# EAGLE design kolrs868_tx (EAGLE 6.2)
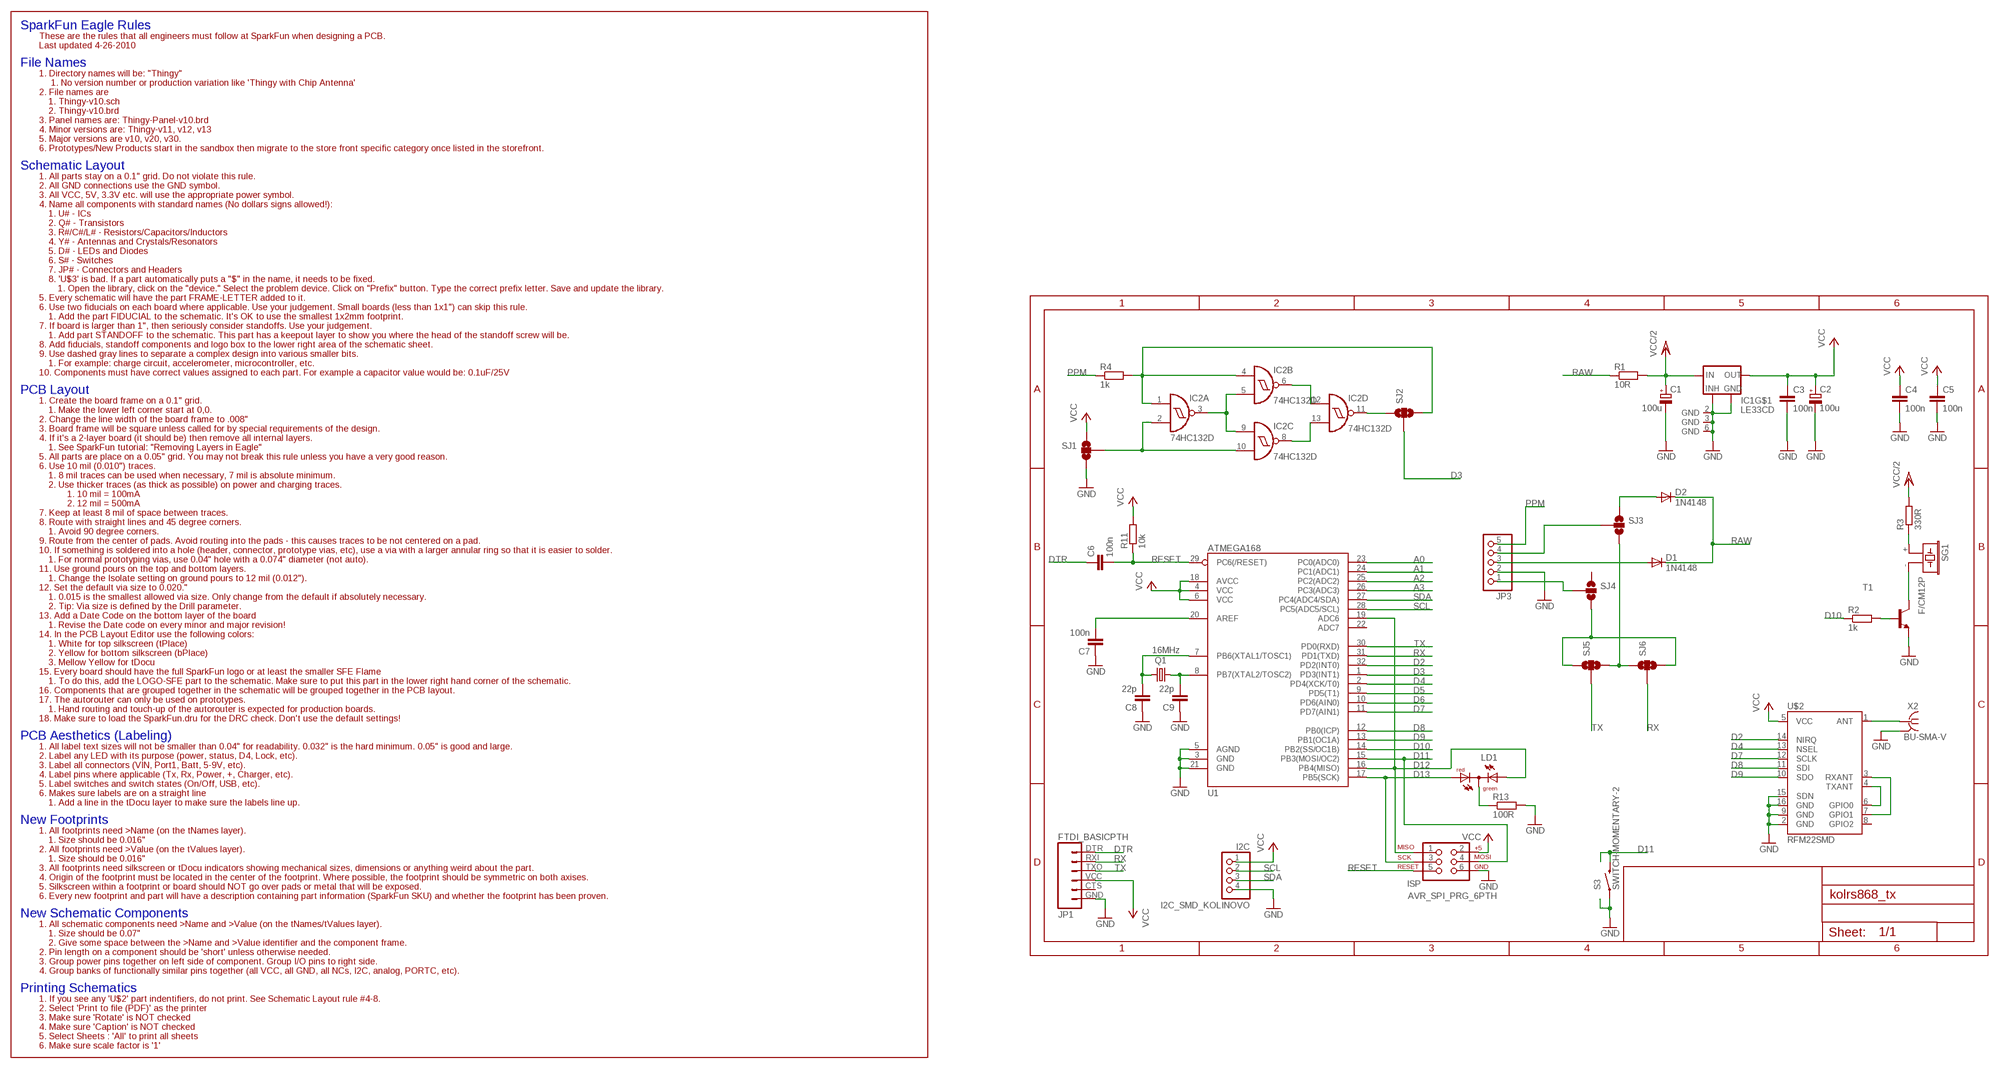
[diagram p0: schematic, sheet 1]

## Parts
C1  100u  CPOL-EUSMCB  [SMC_B]
C2  100u  CPOL-EUSMCB  [SMC_B]
C3  100n  C-EU_KOLIN  [M0805]
C4  100n  C-EU_KOLIN  [M0805]
C5  100n  C-EU_KOLIN  [M0805]
C6  100n  C-EU_KOLIN  [M0805]
C7  100n  C-EU_KOLIN  [M0805]
C8  22p  C-EU_KOLIN  [M0805]
C9  22p  C-EU_KOLIN  [M0805]
D1  1N4148  DIODE-MINIMELF  [MINIMELF]
D2  1N4148  DIODE-MINIMELF  [MINIMELF]
I2C  I2C_SMD_KOLINOVO  [1X04]
IC1  LE33CD  [SO8]
IC2  74HC132D  [SO14]
ISP  AVR_SPI_PRG_6PTH  [2X3]
JP1  FTDI_BASICPTH  [FTDI_BASIC]
JP3  PINHD-1X5  [1X05]
LD1  DUOLED-RG-C  [DUOLED-C-5MM]
Q1  16MHz  CRYSTALHC49UP  [HC49UP]
R1  10R  R-EU_KOLINM0805  [M0805]
R2  1k  R-EU_KOLINM0805  [M0805]
R3  330R  R-EU_KOLINM0805  [M0805]
R4  1k  R-EU_KOLINM0805  [M0805]
R11  10k  R-EU_KOLINM0805  [M0805]
R13  100R  R-EU_KOLINM0805  [M0805]
S3  SWITCH-MOMENTARY-2  [TACTILE_SWITCH_TALL]
SG1  F/CM12P  [F/CM12P]
SJ1  SOLDERJUMPER_2WAYS  [SJ_3]
SJ2  SOLDERJUMPER_2WAYS  [SJ_3]
SJ3  SOLDERJUMPER_2WAYS  [SJ_3]
SJ4  SOLDERJUMPER_2WAYS  [SJ_3]
SJ5  SOLDERJUMPER_2WAYS  [SJ_3]
SJ6  SOLDERJUMPER_2WAYS  [SJ_3]
T1  BC848-NPN-SOT23-BEC  [SOT23-BEC]
U1  ATMEGA168  [TQFP32-08]
U$2  RFM22SMD  [RFM22-XXX-S2]
X2  BU-SMA-V  [BU-SMA-V]

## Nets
A0: U1.23(PC0(ADC0))
A1: U1.24(PC1(ADC1))
A2: U1.25(PC2(ADC2))
A3: U1.26(PC3(ADC3))
D2: U1.32(PD2(INT0)) U$2.14(NIRQ)
D3: SJ2.2 U1.1(PD3(INT1))
D4: U1.2(PD4(XCK/T0)) U$2.13(NSEL)
D5: U1.9(PD5(T1))
D6: U1.10(PD6(AIN0))
D7: U1.11(PD7(AIN1)) U$2.12(SCLK)
D8: U1.12(PB0(ICP)) U$2.11(SDI)
D9: U1.13(PB1(OC1A)) U$2.10(SDO)
D10: R2.1 U1.14(PB2(SS/OC1B))
D11: ISP.4 S3.B2 U1.15(PB3(MOSI/OC2))
D12: ISP.1 LD1.AX(AG) U1.16(PB4(MISO)) U1.19(ADC6)
D13: ISP.3 LD1.AR U1.17(PB5(SCK))
DTR: C6.1 JP1.DTR
GND: C1.- C2.- C3.2 C4.2 C5.2 C7.1 C8.1 C9.1 I2C.4 IC1.2(GND) IC1.3(GND) IC1.5(INHIBIT) IC1.6(GND) IC1.7(GND) ISP.6 JP1.GND JP3.2 R13.2 S3.A2 SJ1.3 T1.E U1.3(GND) U1.5(AGND) U1.21(GND) U$2.2(GND) U$2.9(GND) U$2.15(SDN) U$2.16(GND) X2.2(GND)
N$1: C7.2 U1.20(AREF)
N$2: U$2.4(TXANT) U$2.6(GPIO0)
N$3: U$2.3(RXANT) U$2.7(GPIO1)
N$4: U$2.1(ANT) X2.1
N$5: JP3.1 SJ4.2
N$6: C8.2 Q1.2 U1.7(PB6(XTAL1/TOSC1))
N$7: C9.2 Q1.1 U1.8(PB7(XTAL2/TOSC2))
N$8: LD1.C R13.1
N$10: R2.2 T1.B
N$11: SG1.- T1.C
N$12: R3.1 SG1.+
N$13: D1.A JP3.3
N$14: JP3.4 SJ3.2
N$16: D2.A SJ3.1
N$17: IC2.3(A:O) IC2.5(B:I1) IC2.9(C:I0)
N$18: IC2.11(D:O) SJ2.1
N$19: IC2.2(A:I1) IC2.10(C:I1) SJ1.2
N$20: IC2.8(C:O) IC2.13(D:I1)
N$21: IC2.6(B:O) IC2.12(D:I0)
N$24: IC2.1(A:I0) IC2.4(B:I0) R4.2 SJ2.3
N$25: SJ4.3 SJ5.1 SJ6.3
N$26: SJ3.3 SJ5.3 SJ6.1
PPM: JP3.5 R4.1
RAW: D1.C D2.C R1.1
RESET: C6.2 ISP.5 R11.1 U1.29(PC6(/RESET))
RX: JP1.RXI SJ6.2 U1.31(PD1(TXD))
SCL: I2C.2 U1.28(PC5(ADC5/SCL))
SDA: I2C.3 U1.27(PC4(ADC4/SDA))
TX: JP1.TXO SJ5.2 U1.30(PD0(RXD))
VCC: C2.+ C3.1 C4.1 C5.1 I2C.1 IC1.1(OUT) ISP.2 JP1.VCC R11.2 SJ1.1 U1.4(VCC) U1.6(VCC) U1.18(AVCC) U$2.5(VCC)
VCC/2: C1.+ IC1.8(IN) R1.2 R3.2
Unconnected: JP1.CTS SJ4.1 U1.22(ADC7) U$2.8(GPIO2)

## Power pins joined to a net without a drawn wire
GND: IC2.7(P:GND) X2.3(GND) X2.4(GND) X2.5(GND)
VCC: IC2.14(P:VCC)

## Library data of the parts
C1 C2 = rcl:CPOL-EU: POLARIZED CAPACITOR, European symbol
C3-C9 = PINHEAD_RC:C-EU_KOLIN: CAPACITOR, European symbol
D1 D2 = diode:DIODE-: DIODE
I2C = PINHEAD_RC:I2C_SMD_KOLINOVO: PIN HEADER
IC1 = libstabilizatory:LE33CD: VOLTAGE REGULATOR WITH INHIBIT
IC2 = 74xx-eu:74*132: Quad 2-input NAND schmitt trigger
ISP = SparkFun:AVR_SPI_PRG_6: AVR ISP 6 Pin This is the reduced ISP connector for AVR programming. Common on Arduino. This footprint will take up less PCB space and can be used with a 10-pin to 6-pin adapter such as SKU: BOB-08508
JP1 = SparkFun:FTDI_BASIC: FTDI Basic: 3.3V and 5V
JP3 = pinhead:PINHD-1X5: PIN HEADER
LD1 = led:DUOLED-RG-C: DUO LED 2 colors (red/green), 5 mm, round, common Cathode www.ligitek.com or other producers.
Q1 = crystal:CRYSTAL: CRYSTAL; OC_FARNELL: unknown; OC_NEWARK: unknown
R1-R4 R11 R13 = PINHEAD_RC:R-EU_KOLIN: RESISTOR, European symbol
S3 = SparkFun:SWITCH-MOMENTARY-2
SG1 = buzzer:F/CM12P: BUZZER
SJ1-SJ6 = SparkFun:SOLDERJUMPER_2WAY: Solder Jumper 2 way solder jumper
T1 = transistor:*-NPN-: NPN Transistror BF959 corrected 2008.03.06
U1 = SparkFun:ATMEGA168
U$2 = SparkFun:RFM22: Description: The RFM22 is a low-power, low cost radio that is capable of operating in the 434MHz and 900MHz open bands. It's frequency is software defined and there are some very good libraries written for it.
X2 = con-coax:BU-SMA-V: FEMALE SMA CONNECTOR Radiall distributor RS 112-3794; OC_FARNELL: unknown; OC_NEWARK: unknown

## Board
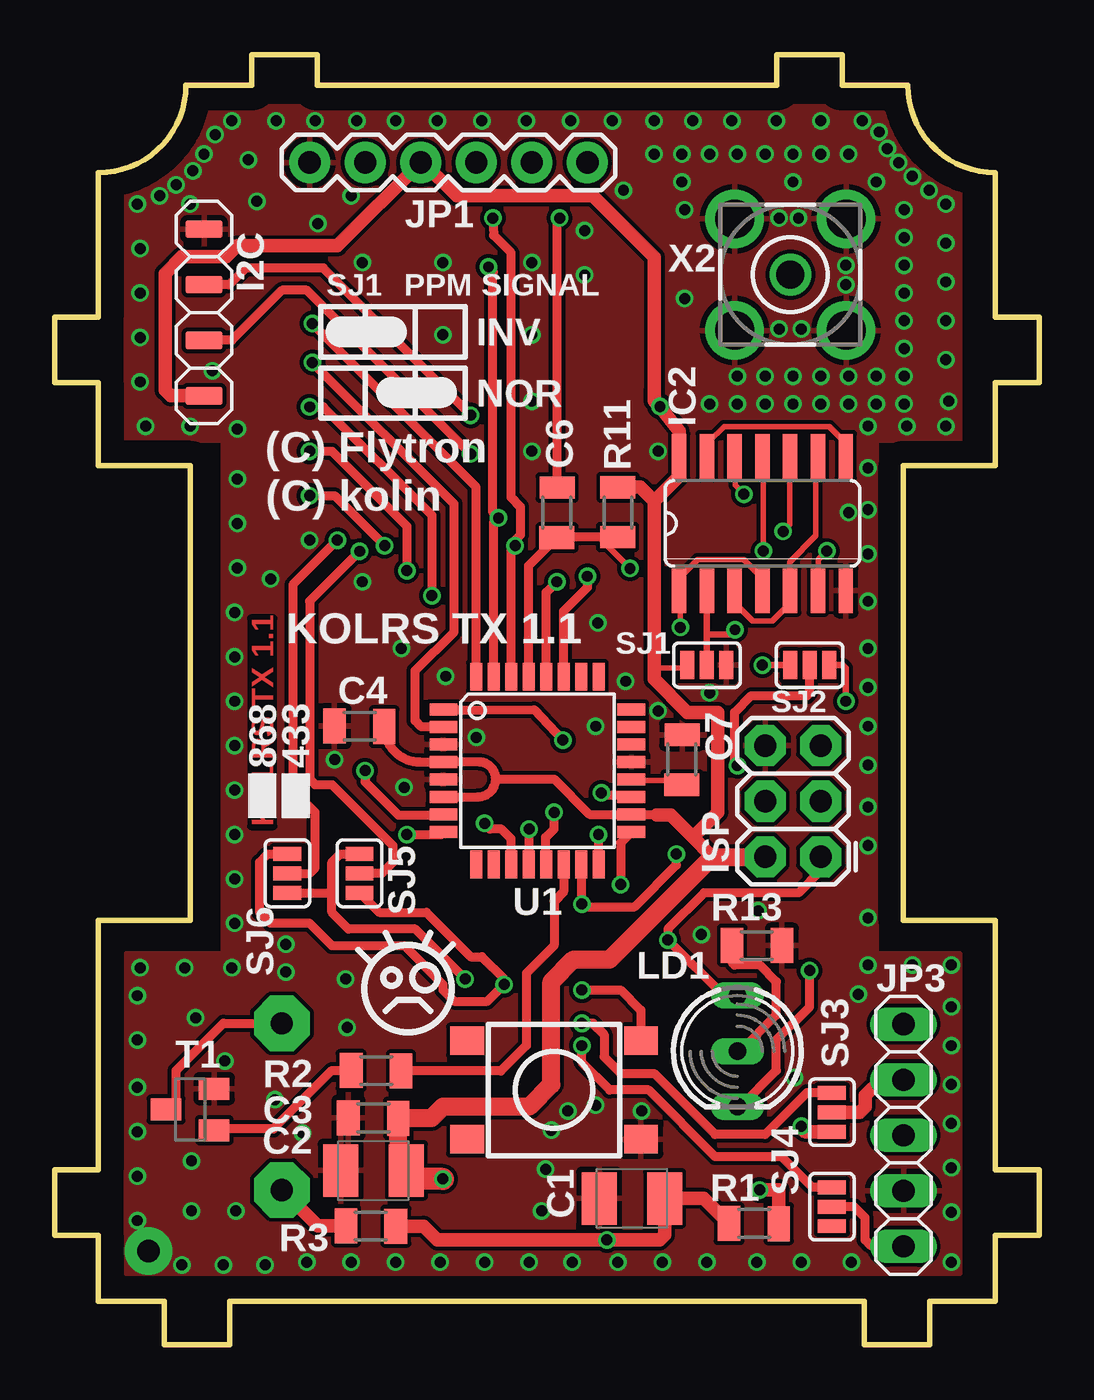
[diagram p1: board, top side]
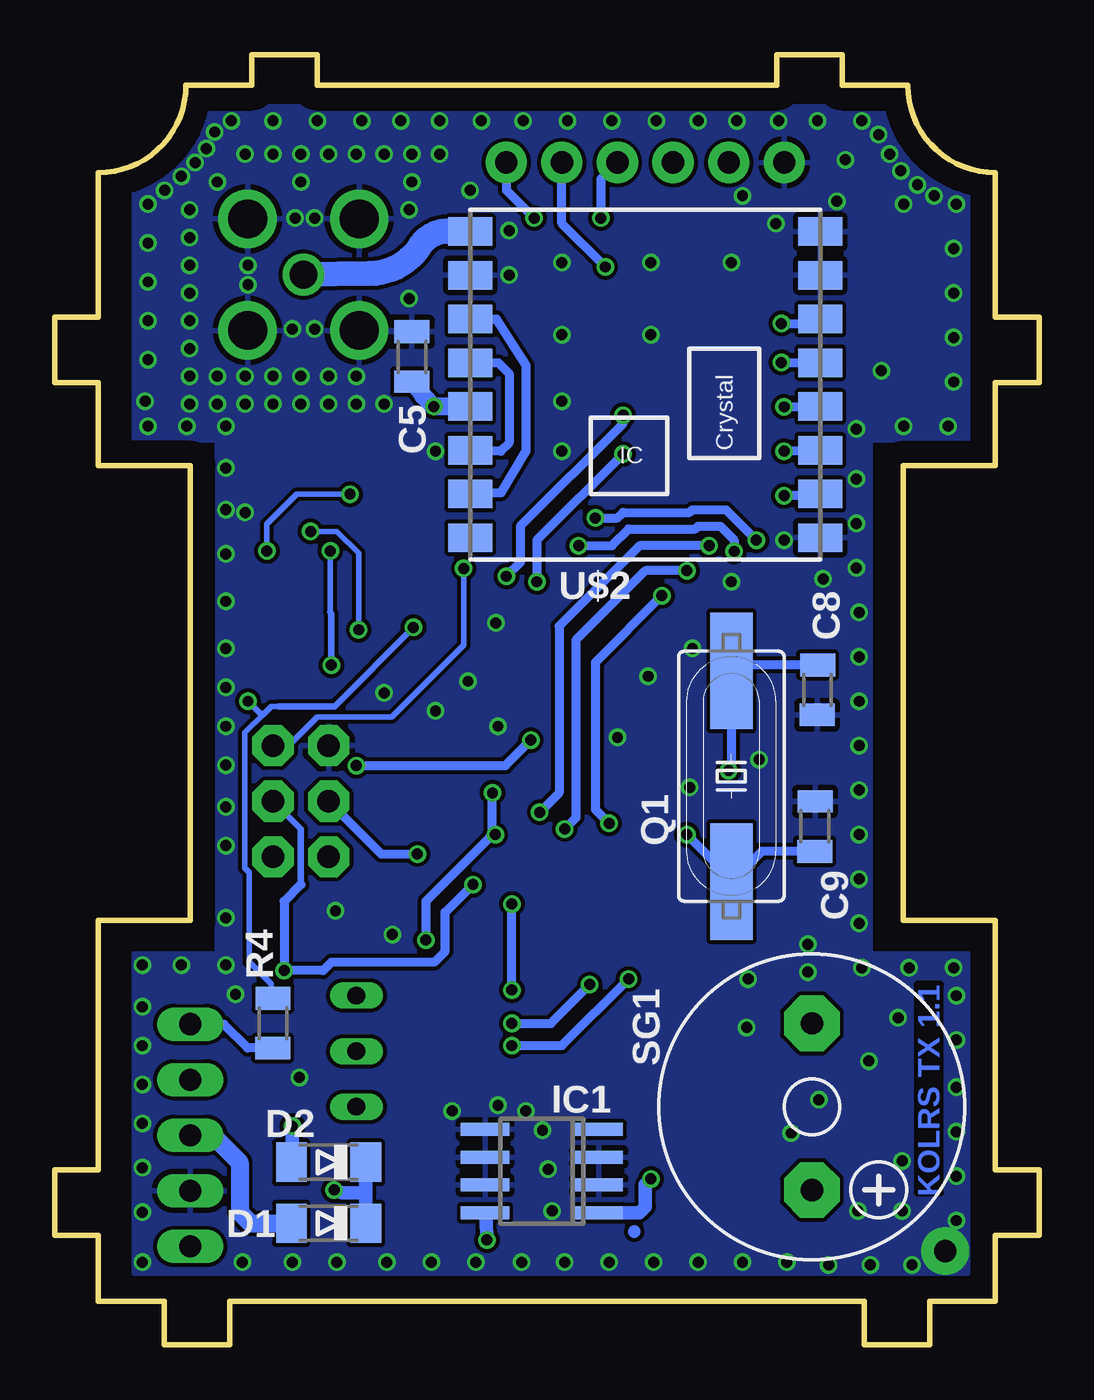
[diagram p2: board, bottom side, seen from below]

Size 45 x 59 mm. Coordinates in mm from the lower left corner, seen from the top.
Outline: 2,2 5,2 5,0 8,0 8,2 37,2 37,0 40,0 40,2 43,2 43,5 45,5 45,8 43,8 43,19.4 38.8,19.4 38.8,40.2 43,40.2 43,44 45,44 45,47 43,47 43,53.6 arc-90 39,57.6 36,57.6 36,59 33,59 33,57.6 12,57.6 12,59 9,59 9,57.6 6,57.6 arc-90 2,53.6 2,47 0,47 0,44 2,44 2,40.2 6.2,40.2 6.2,19.4 2,19.4 2,8 0,8 0,5 2,5 2,2
Copper layers (1*16): Top 0.018mm / dielectric 1.5mm / Bottom 0.018mm
Design rules: minimum track width 0.15mm, minimum drill 0.3mm, track to track 0.18mm, track to pad 0.18mm, pad to pad 0.18mm, via to via 0.18mm, smd to smd 0.18mm, copper to edge 40mil, drill to drill 8mil, minimum pad ring 0.15mm, minimum via ring 0.15mm, stop-mask expansion 4mil, vias tented up to drill 0.5mm, thermal gap 10mil

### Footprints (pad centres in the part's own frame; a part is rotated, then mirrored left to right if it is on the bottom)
SMC_B = smd 1.6 x 2.4: + -1.5,0; - 1.5,0
M0805 = smd 1.021 x 1.6: 1 -1.131,0.017 | smd 1.046 x 1.6: 2 1.148,0
MINIMELF = smd 1.4 x 1.8: A 1.7,0; C -1.7,0
1X04 = smd 0.813 x 1.676: 1 -3.81,0; 2 -1.27,0; 3 1.27,0; 4 3.81,0
SO8 = smd 0.6 x 2.2: 1 -1.905,-2.6; 2 -0.635,-2.6; 3 0.635,-2.6; 4 1.905,-2.6; 5 1.905,2.6; 6 0.635,2.6; 7 -0.635,2.6; 8 -1.905,2.6
SO14 = smd 0.66 x 2.032: 1 -3.81,-3.073; 2 -2.54,-3.073; 3 -1.27,-3.073; 4 0,-3.073; 5 1.27,-3.073; 6 2.54,-3.073; 7 3.81,-3.073; 8 3.81,3.073; 9 2.54,3.073; 10 1.27,3.073; 11 0,3.073; 12 -1.27,3.073; 13 -2.54,3.073; 14 -3.81,3.073
2X3 = drill 1.016 pad 1.88 octagon: 1 0,0; 2 0,2.54; 3 2.54,0; 4 2.54,2.54; 5 5.08,0; 6 5.08,2.54
FTDI_BASIC = drill 1.016 pad 1.88: CTS 10.16,0; DTR 0,0; GND 12.7,0; RXI 2.54,0; TXO 5.08,0; VCC 7.62,0
1X05 = drill 1.016 long: 1 -5.08,0; 2 -2.54,0; 3 0,0; 4 2.54,0; 5 5.08,0
DUOLED-C-5MM = drill 0.813 long: AR 2.54,0; AX -2.54,0; C 0,0
HC49UP = smd 5.334 x 1.93: 1 -4.826,0; 2 4.826,0
TACTILE_SWITCH_TALL = smd 1.55 x 1.3: A1 -3.975,-2.25; A2 3.975,-2.25; B1 -3.975,2.25; B2 3.975,2.25
F/CM12P = drill 1.016 pad 2.54 octagon: + 3.81,0; - -3.81,0
SJ_3 = smd 0.635 x 1.27: 1 -0.889,0; 2 0,0; 3 0.889,0
SOT23-BEC = smd 1 x 1.4: B -0.95,-1.1; C 0,1.1; E 0.95,-1.1
TQFP32-08 = smd 1.27 x 0.559: 1 -4.293,2.8; 2 -4.293,2; 3 -4.293,1.2; 4 -4.293,0.4; 5 -4.293,-0.4; 6 -4.293,-1.2; 7 -4.293,-2; 8 -4.293,-2.8; 17 4.293,-2.8; 18 4.293,-2; 19 4.293,-1.2; 20 4.293,-0.4; 21 4.293,0.4; 22 4.293,1.2; 23 4.293,2; 24 4.293,2.8 | smd 0.559 x 1.27: 9 -2.8,-4.293; 10 -2,-4.293; 11 -1.2,-4.293; 12 -0.4,-4.293; 13 0.4,-4.293; 14 1.2,-4.293; 15 2,-4.293; 16 2.8,-4.293; 25 2.8,4.293; 26 2,4.293; 27 1.2,4.293; 28 0.4,4.293; 29 -0.4,4.293; 30 -1.2,4.293; 31 -2,4.293; 32 -2.8,4.293
RFM22-XXX-S2 = smd 2 x 1.3: 1 -8,7; 2 -8,5; 3 -8,3; 4 -8,1; 5 -8,-1; 6 -8,-3; 7 -8,-5; 8 -8,-7; 9 8,-7; 10 8,-5; 11 8,-3; 12 8,-1; 13 8,1; 14 8,3; 15 8,5; 16 8,7
BU-SMA-V = drill 1.27: 1 0,0 | drill 1.778: 2 -2.55,2.55; 3 2.55,2.55; 4 2.55,-2.55; 5 -2.55,-2.55

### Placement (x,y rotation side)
C1  26.38,6.7 180 top
C2  14.57,7.97 180 top
C3  14.57,10.38 180 top
C4  13.94,28.29 180 top
C5  28.67,45.18 90 bottom
C6  22.95,38.07 270 top
C7  28.67,26.77 270 top
C8  10.13,29.94 90 bottom
C9  10.26,23.72 270 bottom
D1  32.48,5.56 180 bottom
D2  32.48,8.35 180 bottom
I2C  6.83,47.21 90 top
IC1  22.73,7.94 90 bottom
IC2  32.35,37.56 0 top
ISP  35.02,22.32 90 top
JP1  24.35,54.07 180 top
JP3  38.81,9.58 90 top
LD1  31.21,13.43 270 top
Q1  14.06,26 90 bottom
R1  31.97,5.56 180 top
R2  14.7,12.54 180 top
R3  14.45,5.43 0 top
R4  35.02,14.7 90 bottom
R11  25.75,38.07 90 top
R13  32.1,18.26 0 top
S3  22.83,11.65 0 top
SG1  10.38,10.89 270 bottom
SJ1  29.81,31.08 0 top
SJ2  34.51,31.08 0 top
SJ3  35.53,10.64 90 top
SJ4  35.53,6.32 90 top
SJ5  13.94,21.56 270 top
SJ6  10.64,21.56 270 top
T1  6.19,10.76 90 top
U1  22.07,26.26 0 top
U$2  18,43.91 0 bottom
X2  33.63,48.94 0 top

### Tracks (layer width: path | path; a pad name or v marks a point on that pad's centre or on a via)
D2  (via drill 0.5)
  Top 0.406: U1.32 19.27,39.22 v11.78,46.7
  Bottom 0.406: v11.78,46.7 9.45,46.7 U$2.14
D3  (via drill 0.5)
  Top 0.406: v23.23,27.65 21.91,29.05 19.65,29.03 18.51,29.03 18.48,29.05 U1.1 | v31.21,26.49 31.11,26.49 31.03,26.56 31.08,26.61 31.08,28.92 31.84,29.69 34.38,29.69 34.51,29.81 SJ2.2
  Bottom 0.406: v23.23,27.65 24.4,26.49 v31.21,26.49
D4  (via drill 0.5)
  Top 0.406: U1.2 16.76,28.26 16.48,28.54 16.48,30.83 18.26,32.61 18.26,38.45 v11.78,44.93
  Bottom 0.406: v11.78,44.93 9.26,44.93 U$2.13
D7  (via drill 0.5)
  Top 0.406: v11.65,42.89 12.29,42.89 17.24,37.94 v17.24,34.26 | U1.11 20.87,23.14 20.41,23.59 19.91,23.59 v19.65,23.84
  Bottom 0.406: U$2.12 10.14,42.77 10.27,42.89 v11.65,42.89 | v19.65,23.84 20.29,24.48 20.29,31.21 v17.24,34.26
D8  (via drill 0.5)
  Top 0.406: v11.65,40.86 12.67,40.86 16.1,37.43 v16.1,35.4 | U1.12 21.68,21.98 v21.68,23.59
  Bottom 0.406: U$2.11 10.05,40.86 v11.65,40.86 | v16.1,35.4 18,35.4 21.18,32.23 21.18,24.1 v21.68,23.59
D9  (via drill 0.5)
  Top 0.406: v11.65,38.83 12.79,38.83 v15.08,36.54 | U1.13 22.45,21.98 22.45,23.21 22.83,23.59 v22.83,24.35
  Bottom 0.406: U$2.10 10.08,38.83 v11.65,38.83 | v15.08,36.54 18.26,36.54 21.94,32.86 21.94,25.24 v22.83,24.35
D10
  Top 0.406: U1.14 23.27,20.73 22.83,20.29 22.83,18.26 21.56,16.99 21.56,13.68 20.4,12.52 R2.1
D11  (via drill 0.5)
  Top 0.406: U1.15 24.1,21.94 v24.1,20.16 24.23,20.03 26.51,20.03 28.42,21.94 v28.42,22.45 | v24.1,16.22 25.88,16.22 26.8,15.3 S3.B2
  Bottom 0.406: v24.1,16.22 v24.1,20.16 | v28.42,22.45 30.07,22.45 ISP.4
D12  (via drill 0.5)
  Top 0.406: U1.19 26.26,25.11 24.99,25.11 v24.99,25.24 | v24.86,23.34 24.86,22.07 U1.16 | LD1.AX 30.57,15.97 v28.04,18.51 28.04,19.02 29.69,20.67 34,20.67 35.02,21.68 ISP.1
  Bottom 0.406: v24.99,25.24 24.99,23.34 v24.86,23.34 25.11,23.21 28.04,20.29 v28.04,18.51
D13  (via drill 0.5)
  Top 0.406: LD1.AR 31.34,10.89 32.99,12.54 32.99,13.94 34.51,15.46 v34.51,17.11 | v25.88,21.05 25.88,22.95 26.26,23.34 U1.17
  Bottom 0.305: 33.75,21.05 33.75,23.59 ISP.3
  Bottom 0.406: v25.88,21.05 27.15,19.78 27.15,18 27.65,17.49 32.35,17.49 32.73,17.11 v34.51,17.11 34.51,20.29 33.75,21.05
DTR  (via drill 0.5)
  Top 0.406: C6.1 22.97,51.42 v23.08,51.53
  Bottom 0.406: v23.08,51.53 24.35,52.8 JP1.DTR
GND  (via drill 0.5, 1.02 pad 2.18)
  other vias: 4.79,52.55 27.4,55.98 36.92,55.98 40.73,52.16 40.73,42.01 37.18,30.07 37.18,17.37 40.99,17.37 40.99,3.78 3.91,17.24 15.97,25.5 13.3,16.73 17.75,49.5 26,52.8 36.29,38.07 27.4,54.45 40.73,50.39 40.73,48.61 40.73,46.83 40.73,45.05 40.86,43.15 38.96,42.01 33.11,46.45 34.13,46.45 36.16,48.48 36.16,49.37 34,51.53 33.11,51.53 28.8,51.91 37.18,42.01 37.18,40.1 37.18,38.2 37.18,36.16 37.18,34 37.18,31.84 37.18,28.29 37.18,26.51 37.18,24.61 29.56,18.76 39.21,17.37 40.99,15.46 40.99,13.68 40.99,11.91 40.99,10.13 40.99,8.1 40.99,6.06 36.42,3.78 34.13,3.78 32.1,3.78 29.81,3.78 27.78,3.78 9.62,3.65 7.71,3.65 5.81,3.65 3.78,5.68 3.78,7.71 3.78,9.75 3.78,11.78 3.78,13.94 3.78,15.97 5.94,17.24 8.1,17.24 8.22,19.27 8.22,21.3 8.22,23.34 8.22,25.37 8.22,27.4 8.22,29.43 8.22,31.46 8.22,33.5 6.19,42.01 3.78,52.16 5.56,53.05 6.32,53.69 6.83,54.45 7.33,55.34 8.1,55.98 10.13,55.98 11.91,55.98 13.81,55.98 15.59,55.98 17.49,55.98 29.18,55.98 30.96,55.98 32.99,55.98 35.02,55.98 37.69,55.47 38.07,54.7 38.58,54.07 39.21,53.44 39.97,52.8 6.19,52.16 9.24,52.29 12.03,51.28 13.56,52.55 8.86,54.2 28.67,54.45 29.94,54.45 31.21,54.45 32.48,54.45 33.75,54.45 35.02,54.45 36.29,54.45 37.56,53.18 38.83,51.91 38.83,50.64 38.83,49.37 38.83,48.1 38.83,46.83 38.83,45.56 38.83,44.29 37.56,44.29 35.02,44.29 36.29,44.29 33.75,44.29 32.48,44.29 31.21,44.29 29.94,43.02 31.21,43.02 32.48,43.02 33.75,43.02 35.02,43.02 36.29,43.02 37.56,43.02 38.83,43.02 28.67,53.18 33.75,53.18 14.06,49.5 17.75,46.2 21.81,49.5 21.81,46.2 21.81,43.15 21.81,40.86 27.59,40.86 22.45,8.03 11.65,36.8 9.87,35.02 7.21,44.55 12.79,26.77 15.84,31.84 17.88,30.57 26.1,30.35 24.73,28.29 14.06,34.89 19.27,27.78 27.59,28.99 32.16,19.84 10.57,18.32 10.57,17.05 13.37,14.51 33.81,12.22 22.26,6.13 26.83,10.7 11.33,9.68 8.29,6.13 6.25,6.13 7.78,12.99 36.73,16.03 10.06,11.21 4.29,4.29 19.53,55.98 21.56,55.98 23.59,55.98 25.5,55.98 4.16,42.01 3.91,44.04 3.91,46.07 3.91,48.1 3.91,50.13 8.35,35.53 8.35,37.56 8.35,39.59 8.35,41.88 37.18,22.83 37.18,19.53 25.75,3.78 21.68,3.78 19.65,3.78 17.62,3.78 15.59,3.78 13.56,3.78 11.53,3.78 23.65,3.78 6.45,14.95 6.25,8.41 24.23,50.96 24.23,48.93 28.8,47.85 24.83,33.01 22.7,9.81 24.73,10.95 23.46,10.7 29.94,29.81
  pour Bottom: 3.27,3.27 41.37,3.27 41.37,17.88 37.56,17.88 37.56,41.37 41.37,41.37 41.37,52.8 37.56,56.61 7.08,56.61 3.27,52.8 3.27,41.37 7.71,41.37 7.71,17.88 3.27,17.88
  pour Top: 3.27,3.27 41.37,3.27 41.37,17.88 37.56,17.88 37.56,41.37 41.37,41.37 41.37,52.8 37.56,56.61 7.08,56.61 3.27,52.8 3.27,41.37 7.71,41.37 7.71,17.88 3.27,17.88
N$1
  Top 0.254: U1.20 26.4,25.8 28.5,25.8 28.6,25.7 C7.2
N$2
  Bottom 0.406: U$2.4 24.72,44.91 24.23,44.42 24.23,41.24 24.61,40.86 25.19,40.86 U$2.6
N$3
  Bottom 0.406: U$2.3 24.81,46.91 23.46,44.8 23.46,40.86 24.61,38.96 25.19,38.96 U$2.7
N$4
  Bottom 0.61: U$2.1 26.77,50.9
  Bottom 1.143: X2.1 30.57,48.99 arc-56 28.29,50.26
  Bottom 1.151: 26.77,50.9 arc-69 28.29,50.26
N$5
  Top 0.406: JP3.1 38.77,4.54 37.31,4.54 37.05,4.79 37.05,5.81 36.54,6.32 SJ4.2
N$6  (via drill 0.5)
  Top 0.406: v14.19,26.26 14.19,25.75 15.72,24.23 17.74,24.23 U1.7
  Bottom 0.406: C8.2 13.81,31.09 Q1.2 14.06,26.38 v14.19,26.26
N$7  (via drill 0.5)
  Top 0.406: v16.1,23.34 17.65,23.34 U1.8
  Bottom 0.406: C9.2 12.67,22.57 Q1.1 14.06,21.3 v16.1,23.34
N$8
  Top 0.406: LD1.C 31.34,13.43 32.99,15.08 32.99,16.61 32.23,17.37 31.08,17.37 30.96,17.49 30.96,18.26 R13.1
N$10
  Top 0.406: T1.B 7.33,9.87 10,9.87 12.67,12.54 R2.2
N$11
  Top 0.406: SG1.- 7.71,14.7 5.56,12.54 5.56,10.76 T1.C
N$12
  Top 0.61: SG1.+ 12.02,5.45 R3.1
N$13
  Bottom 0.813: JP3.3 37.78,9.58 36.54,8.35 36.54,6.06 36.04,5.56 D1.A
N$14
  Top 0.61: SJ3.2 36.8,10.64 37.05,10.89 37.05,11.4 37.78,12.12 JP3.4
N$16  (via drill 0.5)
  Top 0.61: SJ3.1 34.38,9.75 arc-90 v34.13,10
  Bottom 0.406: 34.13,9.19 D2.A
  Bottom 0.61: v34.13,10 34.13,8.4 arc90 D2.A
N$17
  Top 0.254: IC2.3 31.1,34.4 31.1,33.9 31.9,33.1 32.8,33.1 33.6,33.9 33.6,34.4 IC2.5 33.6,34.6 33.6,35.8 34.8,37 34.8,40.6 IC2.9
N$18  (via drill 0.5)
  Top 0.254: v32.4,36.3 32.4,40.6 IC2.11
  Top 0.305: v32.35,31.08 SJ2.1
  Bottom 0.254: 32.4,33.5 v32.4,36.3
  Bottom 0.305: 32.4,33.5 32.35,33.45 v32.35,31.08
N$19  (via drill 0.5)
  Top 0.254: 29.9,34.4 IC2.2 | v33.3,37.2 33.6,37.5 33.6,40.6 IC2.10 | v31.1,32.7 30.88,32.48
  Top 0.305: SJ1.2 29.81,32.48 | 29.81,32.48 IC2.2 | 30.88,32.48 29.81,32.48
  Bottom 0.254: v33.3,37.2 32.1,37.2 31.1,36.2 v31.1,32.7
N$20
  Top 0.254: IC2.13 29.9,40.7 29.9,41.3 30.6,42 35.4,42 36.1,41.3 36.1,40.7 IC2.8
N$21  (via drill 0.5)
  Top 0.254: v35.3,36.3 34.9,35.9 IC2.6 | v31.5,38.9 31.12,39.31 31.1,40.6 IC2.12
  Bottom 0.254: v31.5,38.9 33.93,38.9 35.3,37.53 v35.3,36.3
N$24  (via drill 0.5)
  Top 0.254: IC2.4 32.3,34.5 32.3,35.1 31.5,35.9 29.4,35.9 28.6,35.1 28.6,34.5 IC2.1 28.6,34.4 v28.6,32.81
  Top 0.305: SJ2.3 36.04,31.08 36.16,30.96 v36.16,29.43
  Bottom 0.254: 34.77,29.2 35.1,29.2 35.45,28.85 36.3,28 36.3,21.8 36.1,21.6 36.1,17.5 35.1,16.5 35.1,15.9 R4.2
  Bottom 0.305: v36.16,29.43 35.58,28.85 35.45,28.85 | v28.6,32.81 32.21,29.2 34.77,29.2
N$25  (via drill 0.5)
  Top 0.406: SJ4.3 34.64,7.21 33.24,8.6 30.19,8.6 27.15,11.65 25.37,11.65 24.1,12.92 v24.1,13.68 | SJ6.3 12.67,20.67 | v18.76,16.73 16.48,19.02 13.43,19.02 12.67,19.78 12.67,20.67 | 12.67,20.67 12.67,22.07 13.05,22.45 SJ5.1
  Bottom 0.406: v24.1,13.68 21.81,13.68 v18.76,16.73
N$26  (via drill 0.5)
  Top 0.406: SJ3.3 34.38,11.53 32.48,9.62 30.19,9.62 27.4,12.41 25.88,12.41 25.11,13.18 25.11,14.19 24.61,14.7 v24.1,14.7 | SJ6.1 9.75,22.45 9.37,22.07 9.37,19.78 9.87,19.27 11.65,19.27 12.67,18.26 15.97,18.26 17.75,16.48 17.75,16.22 18.26,15.72 19.78,15.72 v20.54,16.48 20.54,16.73 19.53,17.75 19.02,17.75 16.99,19.78 14.83,19.78 SJ5.3
  Bottom 0.406: v24.1,14.7 22.32,14.7 v20.54,16.48
PPM
  Bottom 0.406: R4.1 36.17,13.57 37.27,14.66 JP3.5
RAW  (via drill 0.5)
  Top 0.61: R1.1 33.1,7.09 v32.23,7.08
  Bottom 0.61: D1.C 30.78,6.95 | 30.78,6.95 | 30.78,6.95 31.84,6.95 v32.23,7.08 | 30.78,6.95 D2.C
RESET  (via drill 0.5)
  Top 0.254: v26.3,35.5 25,36.8 R11.1
  Top 0.406: U1.29 21.67,35.63 C6.2 22.97,36.94 R11.1
  Bottom 0.254: v26.3,35.5 26.3,32 29.6,28.7 33,28.7 34.3,27.4 35,27.4 ISP.5
RX  (via drill 0.5)
  Top 0.406: 20.07,49.06 v19.83,49.3 20.03,49.3 20.03,38.07 v20.29,37.81 20.07,37.59 U1.31 | SJ6.2 11.65,21.56 11.91,21.81 11.91,24.35 10.89,25.37 10.89,34.77 v12.92,36.8
  Bottom 0.406: 21.56,53.82 JP1.RXI 21.81,51.28 v19.83,49.3 | v20.29,37.81 19.27,37.81 19.02,38.07 15.97,38.07 15.84,38.2 14.32,38.2 v12.92,36.8
SCL  (via drill 0.5)
  Top 0.406: U1.28 22.47,34.4 v22.95,34.89 | v19.02,40.73 11.53,48.23 10.38,48.23 8.1,45.94 I2C.2
  Bottom 0.406: v19.02,40.73 22.95,36.8 v22.95,34.89
SDA  (via drill 0.5)
  Top 0.406: U1.27 23.27,33.55 24.35,34.64 v24.35,35.15 | v19.02,42.51 12.29,49.24 8.73,49.24 7.97,48.48 I2C.3
  Bottom 0.406: v19.02,42.51 19.02,42.13 23.72,37.43 23.72,35.78 v24.35,35.15
TX  (via drill 0.5)
  Top 0.406: v20.03,51.53 20.07,50.74 20.87,49.94 20.87,38.76 21.3,38.32 21.3,37.05 21.05,36.8 v21.05,36.54 20.87,36.36 U1.30 | v13.94,36.29 11.65,34 11.65,25.88 11.91,25.62 12.67,25.62 15.46,22.83 15.46,22.07 14.95,21.56 SJ5.2
  Bottom 0.406: v20.03,51.53 20.03,53.31 JP1.TXO | v21.05,36.54 19.53,36.54 18.76,37.31 15.72,37.31 15.59,37.43 14.57,37.43 13.94,36.8 v13.94,36.29
VCC  (via drill 0.5)
  Top 0.254: SJ1.1 28.8,30.96 27.4,30.96
  Top 0.406: C4.1 arc90 16.68,26.66 U1.4 19.38,26.66 arc-90 20.16,25.88 | 27.53,24.23 27.5,24.26 U1.18 24.45,24.26 22.83,25.88 20.16,25.88 | U1.6 19.34,25.06 arc90 20.16,25.88
  Top 0.61: 27.53,24.23 28.16,24.23 29.11,23.27 | 29.11,23.27 30.07,22.32 | 29.11,23.27 29.24,23.27 30.32,24.35 30.32,28.92 28.92,28.92 27.4,30.45 27.4,30.96 27.4,38.58 | 27.4,38.58 26.76,39.22 R11.2 | 27.4,38.58 28.54,39.72 IC2.14 28.54,41.78 v27.67,42.91 27.4,43.18 27.4,43.66 27.42,49.74 24.61,52.55 18.38,52.55 16.86,54.07 JP1.VCC 12.92,50.26 8.35,50.26 7.84,49.75 5.81,49.75 5.05,48.99 5.05,43.66 5.3,43.4 I2C.1
  Top 0.813: ISP.2 30.07,22.32 25.37,17.62 23.72,17.62 22.7,16.61 22.7,11.91 21.68,10.89 17.75,10.89 17.22,10.37 C3.1 15.7,9.35 C2.+
  Top 1.016: v17.75,7.59 16.45,7.59 C2.+
  Bottom 0.61: IC1.1 18.28,6.04 18,6.32 18,7.33 v17.75,7.59
  Bottom 0.813: U$2.5 v27.67,42.91 28.16,43.4 28.42,43.78 C5.1
VCC/2  (via drill 0.5)
  Top 0.61: R1.2 29.68,6.7 C1.+ 27.88,5.02 27.65,4.79 v25.24,4.79 17.5,4.79 16.86,5.43 R3.2
  Bottom 0.61: v25.24,4.79 25.24,4.92 25.27,5.66 IC1.8
(copper drawn outside any net)
  shapes: Bottom circle x1

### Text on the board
Top: KOLRS TX 1.1
Bottom: KOLRS TX 1.1
tPlace: SJ1 | PPM SIGNAL | INV | NOR | (C) Flytron | (C) kolin | KOLRS TX 1.1 | 868 | 433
